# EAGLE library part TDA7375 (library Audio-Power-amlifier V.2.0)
The TDA7375A is a new technology class AB car radio amplifier able to work either in DUAL BRIDGE or QUAD SINGLE ENDED configuration. The exclusive fully complementary structure of the output stage and the internally fixed gain guarantee the highest power performances with extremely reduced component count. The on board clip detector simplifies gain compression operation. The fault diagnostic makes it possible to detect mistakes during car radio set assembly and wiring in the car.
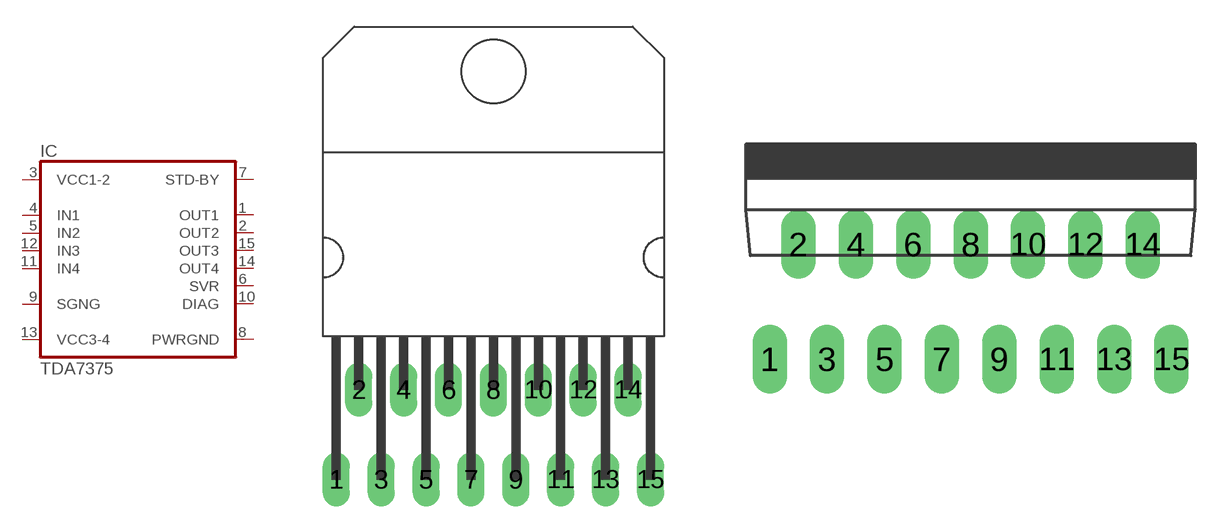
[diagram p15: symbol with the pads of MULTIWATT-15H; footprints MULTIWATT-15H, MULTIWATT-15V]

Designator prefix IC

## TDA7375H  [MULTIWATT-15H]
1  OUT1  out
2  OUT2  out
3  VCC1-2  pwr
4  IN1  in
5  IN2  in
6  SVR  pas
7  STD-BY  in
8  PWRGND  pwr
9  SGNG  pwr
10  DIAG  pas
11  IN4  in
12  IN3  in
13  VCC3-4  pwr
14  OUT4  out
15  OUT3  out

## TDA7375V  [MULTIWATT-15V]
Pads as for MULTIWATT-15H

## Footprint MULTIWATT-15H (pad centres in mm)
Multiwatt 15 horizontal
drill 1.016 long: 1 -8.89,-5.08; 2 -7.62,0; 3 -6.35,-5.08; 4 -5.08,0; 5 -3.81,-5.08; 6 -2.54,0; 7 -1.27,-5.08; 8 0,0; 9 1.27,-5.08; 10 2.54,0; 11 3.81,-5.08; 12 5.08,0; 13 6.35,-5.08; 14 7.62,0; 15 8.89,-5.08

## Footprint MULTIWATT-15V (pad centres in mm)
Multiwatt 15 vertical
drill 1.016 long: 1 -8.89,-5.08; 2 -7.62,0; 3 -6.35,-5.08; 4 -5.08,0; 5 -3.81,-5.08; 6 -2.54,0; 7 -1.27,-5.08; 8 0,0; 9 1.27,-5.08; 10 2.54,0; 11 3.81,-5.08; 12 5.08,0; 13 6.35,-5.08; 14 7.62,0; 15 8.89,-5.08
